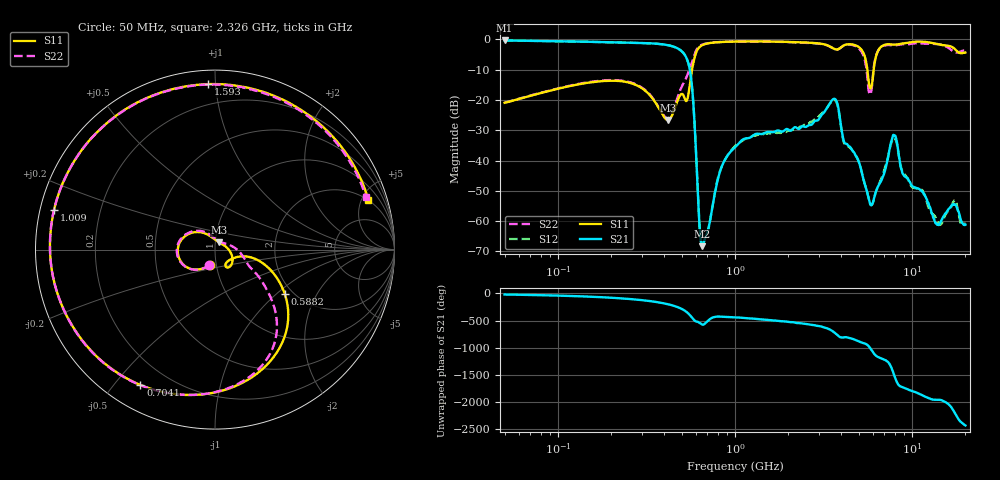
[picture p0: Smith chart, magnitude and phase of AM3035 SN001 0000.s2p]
# Hz S DB R 50
!freq MagS11 AngS11 MagS21 AngS21 MagS12 AngS12 MagS22 AngS22
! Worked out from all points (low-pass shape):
!   1601 points, 50 MHz to 20.05 GHz, reference 50 ohm
!   highest |S21| = -0.34 dB at 50 MHz (marker M1); lowest = -68.3 dB at 653.2 MHz (marker M2)
!   |S21| within 3 dB of the highest: start of sweep to 486.7 MHz
!   lowest |S11| = -26.6 dB at 418.3 MHz (marker M3), VSWR 1.10, Z = 52.2 + j4.24 ohm
!   |S11| at or under -10 dB: start of sweep to 572.4 MHz; 5.602 GHz to 6.081 GHz (478.4 MHz wide, 8.19 % of centre)
!   |S22| runs from -26.0 to -0.7 dB; largest |S21 - S12| = 0.0071
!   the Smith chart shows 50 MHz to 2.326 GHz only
!   S11 on the Smith chart (normalised r, x): 50 MHz: 0.93, -0.16; 588.2 MHz: 1.81, -1.15; 704.1 MHz: 0.10, -0.59; 1.009 GHz: 0.04, +0.12; 1.593 GHz: 0.08, +0.95; 2.326 GHz: 1.95, +5.63
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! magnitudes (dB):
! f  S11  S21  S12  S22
! 50 MHz  -20.9  -0.3  -0.3  -20.8
! 135.9 MHz  -14.6  -0.7  -0.7  -14.5
! 369.6 MHz  -22.4  -1.5  -1.5  -22.2
! 418.3 MHz  -26.6  -1.9  -1.9  -26.0
! 537.6 MHz  -19.9  -6.7  -6.7  -11.9
! 588.2 MHz  -6.7  -25.1  -25.0  -5.5
! 653.2 MHz  -1.9  -68.3  -68.1  -1.7
! 704.1 MHz  -1.3  -63.1  -63.3  -1.2
! 820.9 MHz  -0.9  -43.9  -43.7  -0.9
! 1.005 GHz  -0.7  -35.6  -35.1  -0.7
! 1.009 GHz  -0.7  -35.5  -35.0  -0.7
! 1.593 GHz  -0.7  -30.6  -31.0  -0.7
! 2.326 GHz  -0.9  -29.4  -28.8  -1.0
! 2.722 GHz  -1.1  -28.1  -27.2  -1.2
! 3.701 GHz  -3.3  -19.8  -20.2  -3.3
! 5.032 GHz  -2.6  -40.8  -40.6  -3.0
! 5.89 GHz  -15.9  -54.7  -54.8  -17.2
! 7.402 GHz  -1.6  -37.5  -37.7  -1.8
! 8.008 GHz  -1.7  -31.7  -32.8  -1.9
! 13.84 GHz  -1.5  -61.1  -59.5  -1.5
! 17.39 GHz  -3.1  -54.4  -53.1  -4.2
! 20.05 GHz  -4.4  -61.2  -60.8  -3.6
